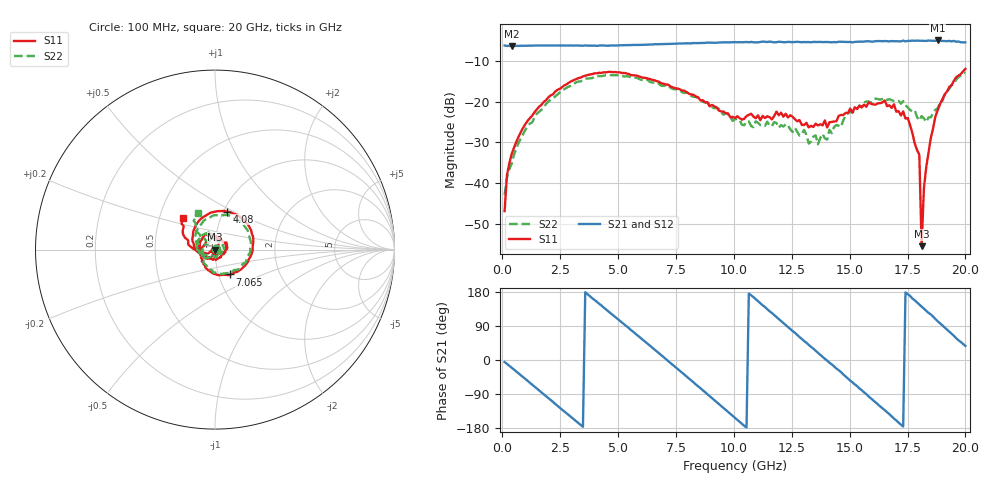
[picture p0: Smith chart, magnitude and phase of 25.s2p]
!Agilent Technologies,N5230C,MY49001569,A.09.33.09
!Agilent N5230C: A.09.33.09
!Date: Monday, July 27, 2015 17:17:14
!Correction: S11(Full 2 Port(1,2))
!S21(Full 2 Port(1,2))
!S12(Full 2 Port(1,2))
!S22(Full 2 Port(1,2))
!S2P File: Measurements: S11, S21, S12, S22:
# Hz S  dB  R 50
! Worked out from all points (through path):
!   201 points, 100 MHz to 20 GHz, reference 50 ohm
!   highest |S21| = -5.01 dB at 18.81 GHz (marker M1); lowest = -6.4 dB at 398.5 MHz (marker M2)
!   group delay of S21, straight-line fit = 145 ps
!   lowest |S11| = -55.4 dB at 18.11 GHz (marker M3), VSWR 1.00, Z = 50.2 + j0.0509 ohm
!   |S11| at or under -10 dB: start of sweep to end of sweep
!   |S22| runs from -42.9 to -12.9 dB; largest |S21 - S12| = 0.021
!   S11 on the Smith chart (normalised r, x): 100 MHz: 1.00, -0.01; 4.08 GHz: 1.04, +0.46; 7.065 GHz: 1.13, -0.32; 20 GHz: 0.66, +0.25
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1e8  -46.86 -63.3  -6.26 -5.3  -6.24 -5.6  -42.88 11.2
1.995e8  -38.09 -45.7  -6.35 -10.1  -6.34 -10.1  -38.71 -52.8
3.985e8  -32.99 -80.1  -6.36 -20.1  -6.36 -20.1  -35.30 -75.3
1.891e9  -19.64 -178.7  -6.25 -95.6  -6.27 -95.8  -20.56 177.4
3.483e9  -13.84 99.6  -6.31 -176.3  -6.30 -176.6  -14.75 97.9
4.08e9  -13.08 72.3  -6.34 153.8  -6.29 153.7  -13.73 70.2
5.3735e9  -13.12 14.6  -6.15 88.7  -6.19 88.5  -13.78 12.9
6.7665e9  -15.13 -45.3  -5.94 17.7  -5.91 17.6  -15.63 -42.9
7.065e9  -15.82 -58.7  -5.92 2.4  -5.90 2.2  -16.08 -56.2
8.7565e9  -20.17 -132.4  -5.61 -84.8  -5.55 -85.0  -20.18 -127.4
1.005e10  -24.06 147.3  -5.45 -152.6  -5.47 -152.4  -24.30 156.8
1.19405e10  -23.37 25.8  -5.33 108.1  -5.38 107.5  -26.40 27.7
1.3433e10  -26.22 -51.4  -5.37 29.8  -5.39 29.0  -28.57 -56.9
1.53235e10  -21.83 -177.9  -5.32 -68.8  -5.22 -68.5  -21.77 -160.3
1.67165e10  -20.92 116.8  -5.25 -142.8  -5.24 -144.0  -19.40 129.9
1.75125e10  -24.03 68.9  -5.11 173.6  -5.11 173.4  -21.44 102.7
1.801e10  -33.03 73.3  -5.08 146.2  -5.18 146.3  -24.62 106.5
1.81095e10  -55.45 17.5  -5.13 140.8  -5.06 140.8  -23.55 108.1
1.8209e10  -41.25 -53.2  -5.15 135.5  -5.14 134.9  -24.10 108.6
1.83085e10  -36.09 -139.4  -5.13 129.5  -5.15 130.0  -25.02 116.6
1.8806e10  -22.08 -167.7  -5.01 101.9  -5.17 102.4  -21.65 132.7
2e10  -11.97 135.6  -5.48 37.2  -5.46 36.3  -12.92 114.5
